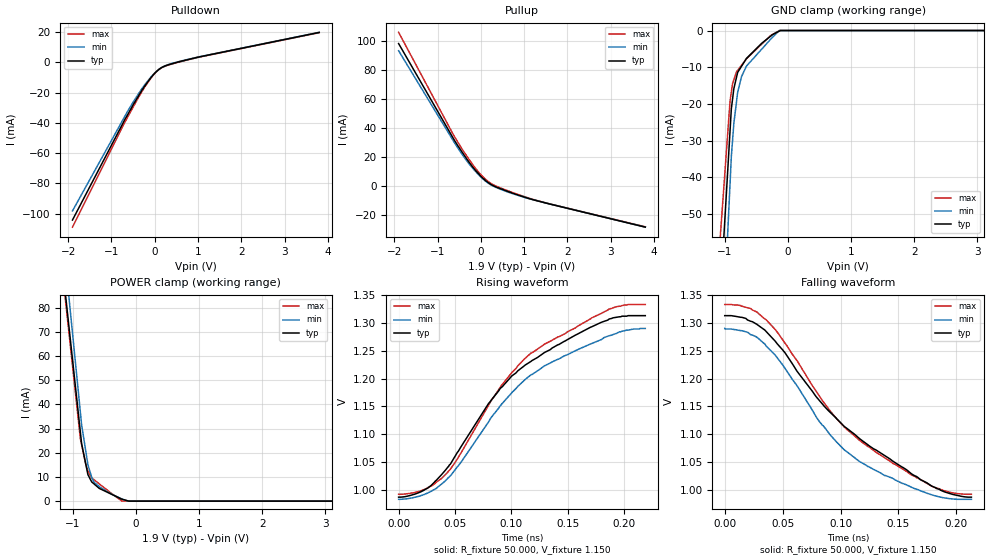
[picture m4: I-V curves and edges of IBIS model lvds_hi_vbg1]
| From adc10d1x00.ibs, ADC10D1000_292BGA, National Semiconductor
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[Model]   lvds_hi_vbg1
Model_type Output
Vref=1.150E+00
Rref=5.000E+01
Cref=0.000E+00
Vmeas=1.150E+00
C_comp   4.84E-13   4.84E-13   4.84E-13
[Voltage Range]   1.900E+00   1.800E+00   2.000E+00
[POWER Clamp Reference]   1.900E+00   1.800E+00   2.000E+00
[GND Clamp Reference]   0.000E+00   0.000E+00   0.000E+00
[Pullup Reference]   1.900E+00   1.800E+00   2.000E+00
[Pulldown Reference]   0.000E+00   0.000E+00   0.000E+00
[Temperature Range]   25   85   -40
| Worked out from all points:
|   slope of the pulldown table from 0 to 0.285 V, typ, clamps not added: 53.7 ohm
|   slope of the pullup table from 0 to 0.285 V, typ, clamps not added: 44.2 ohm
|   GND clamp passes 1 mA (typ) near -0.24 V on its own axis
|   POWER clamp passes 1 mA (typ) near -0.24 V on its own axis
|   rising waveform, R_fixture 50.000, V_fixture 1.150: 20-80 % time 82.7ps typ, 81.7ps min, 78.9ps max; typ from 0.987 V to 1.31 V
|   falling waveform, R_fixture 50.000, V_fixture 1.150: 20-80 % time 93.2ps typ, 73.4ps min, 84.6ps max; typ from 1.31 V to 0.987 V
[GND Clamp]
-2V       -344.8mA   -434.7mA   -277.1mA
-1.8V     -286mA     -361.9mA   -229.3mA
-920mV    -27.26mA   -41.63mA   -19.14mA
-900mV    -21.37mA   -34.35mA   -16.78mA
-880mV    -18.61mA   -29.84mA   -14.42mA
-860mV    -15.84mA   -25.32mA   -13.39mA
-800mV    -11.43mA   -16.88mA   -10.86mA
-740mV    -9.792mA   -12.62mA   -9.504mA
-660mV    -7.601mA   -9.697mA   -7.695mA
-420mV    -3.503mA   -5.11mA    -3.729mA
-140mV    -172uA     0A         0A
4V        0A         0A         0A
[POWER Clamp]
-2.1V     322.7mA    357.6mA    321.9mA
-1.7V     226.3mA    252.5mA    224.9mA
-980mV    52.75mA    63.15mA    50.14mA
-880mV    28.65mA    36.86mA    25.87mA
-860mV    23.83mA    31.6mA     23.38mA
-800mV    16.11mA    21.67mA    15.92mA
-760mV    10.96mA    15.05mA    12.48mA
-700mV    7.94mA     9.824mA    9.618mA
-660mV    7.049mA    7.653mA    8.792mA
-560mV    5.02mA     5.656mA    6.725mA
-220mV    788uA      879.2uA    0A
3.9V      0A         0A         0A
[Pullup]
-1.9V     98.24mA    93.3mA     106mA
-620mV    32.06mA    30.45mA    34.72mA
-380mV    21.12mA    19.68mA    23.21mA
-140mV    11.43mA    10.72mA    12.9mA
23.84nV   6.837mA    6.277mA    7.883mA
180mV     2.218mA    1.847mA    2.93mA
340mV     -407.4uA   -739.1uA   168uA
660mV     -4.075mA   -4.427mA   -3.596mA
1.3V      -10.08mA   -10.13mA   -9.96mA
3.8V      -28.24mA   -28.27mA   -28.04mA
[Pulldown]
-1.9V     -104.2mA   -98.19mA   -108.9mA
-740mV    -40.59mA   -38.24mA   -42.42mA
-520mV    -29.24mA   -27.35mA   -30.73mA
-220mV    -15.29mA   -14.48mA   -15.9mA
-40mV     -8.535mA   -8.276mA   -8.748mA
100mV     -4.671mA   -4.6mA     -4.78mA
320mV     -1.628mA   -1.453mA   -1.823mA
980mV     3.21mA     3.314mA    3.071mA
3.8V      19.7mA     19.77mA    19.52mA
[Rising Waveform]
R_fixture = 50.000
V_fixture = 1.150
V_fixture_min = 1.150
V_fixture_max = 1.150
|  time   V(typ)   V(min)   V(max)
0s        987.2mV    983.3mV    992.4mV
25.5ps    1.003V     994.5mV    1.004V
45ps      1.045V     1.024V     1.035V
80ps      1.156V     1.123V     1.153V
90ps      1.182V     1.151V     1.184V
100.5ps   1.205V     1.175V     1.211V
117.5ps   1.231V     1.207V     1.246V
147ps     1.267V     1.241V     1.28V
186.8ps   1.307V     1.277V     1.325V
218.7ps   1.313V     1.29V      1.333V
[Falling Waveform]
R_fixture = 50.000
V_fixture = 1.150
V_fixture_min = 1.150
V_fixture_max = 1.150
|  time   V(typ)   V(min)   V(max)
0s        1.313V     1.29V      1.333V
20ps      1.305V     1.283V     1.327V
36ps      1.284V     1.258V     1.305V
50.25ps   1.251V     1.224V     1.269V
82ps      1.16V      1.122V     1.168V
95.75ps   1.13V      1.088V     1.13V
116.5ps   1.092V     1.051V     1.089V
138ps     1.062V     1.026V     1.058V
178.8ps   1.007V     991.4mV    1.007V
213ps     987.2mV    983.3mV    992.4mV
[Ramp]
dV/dt_r   1.7621E+00/8.3440E-11   1.7023E+00/8.1710E-11   1.8231E+00/7.8840E-11
dV/dt_f   1.7621E+00/9.3383E-11   1.7023E+00/7.2969E-11   1.8231E+00/8.4250E-11
R_load = 50
